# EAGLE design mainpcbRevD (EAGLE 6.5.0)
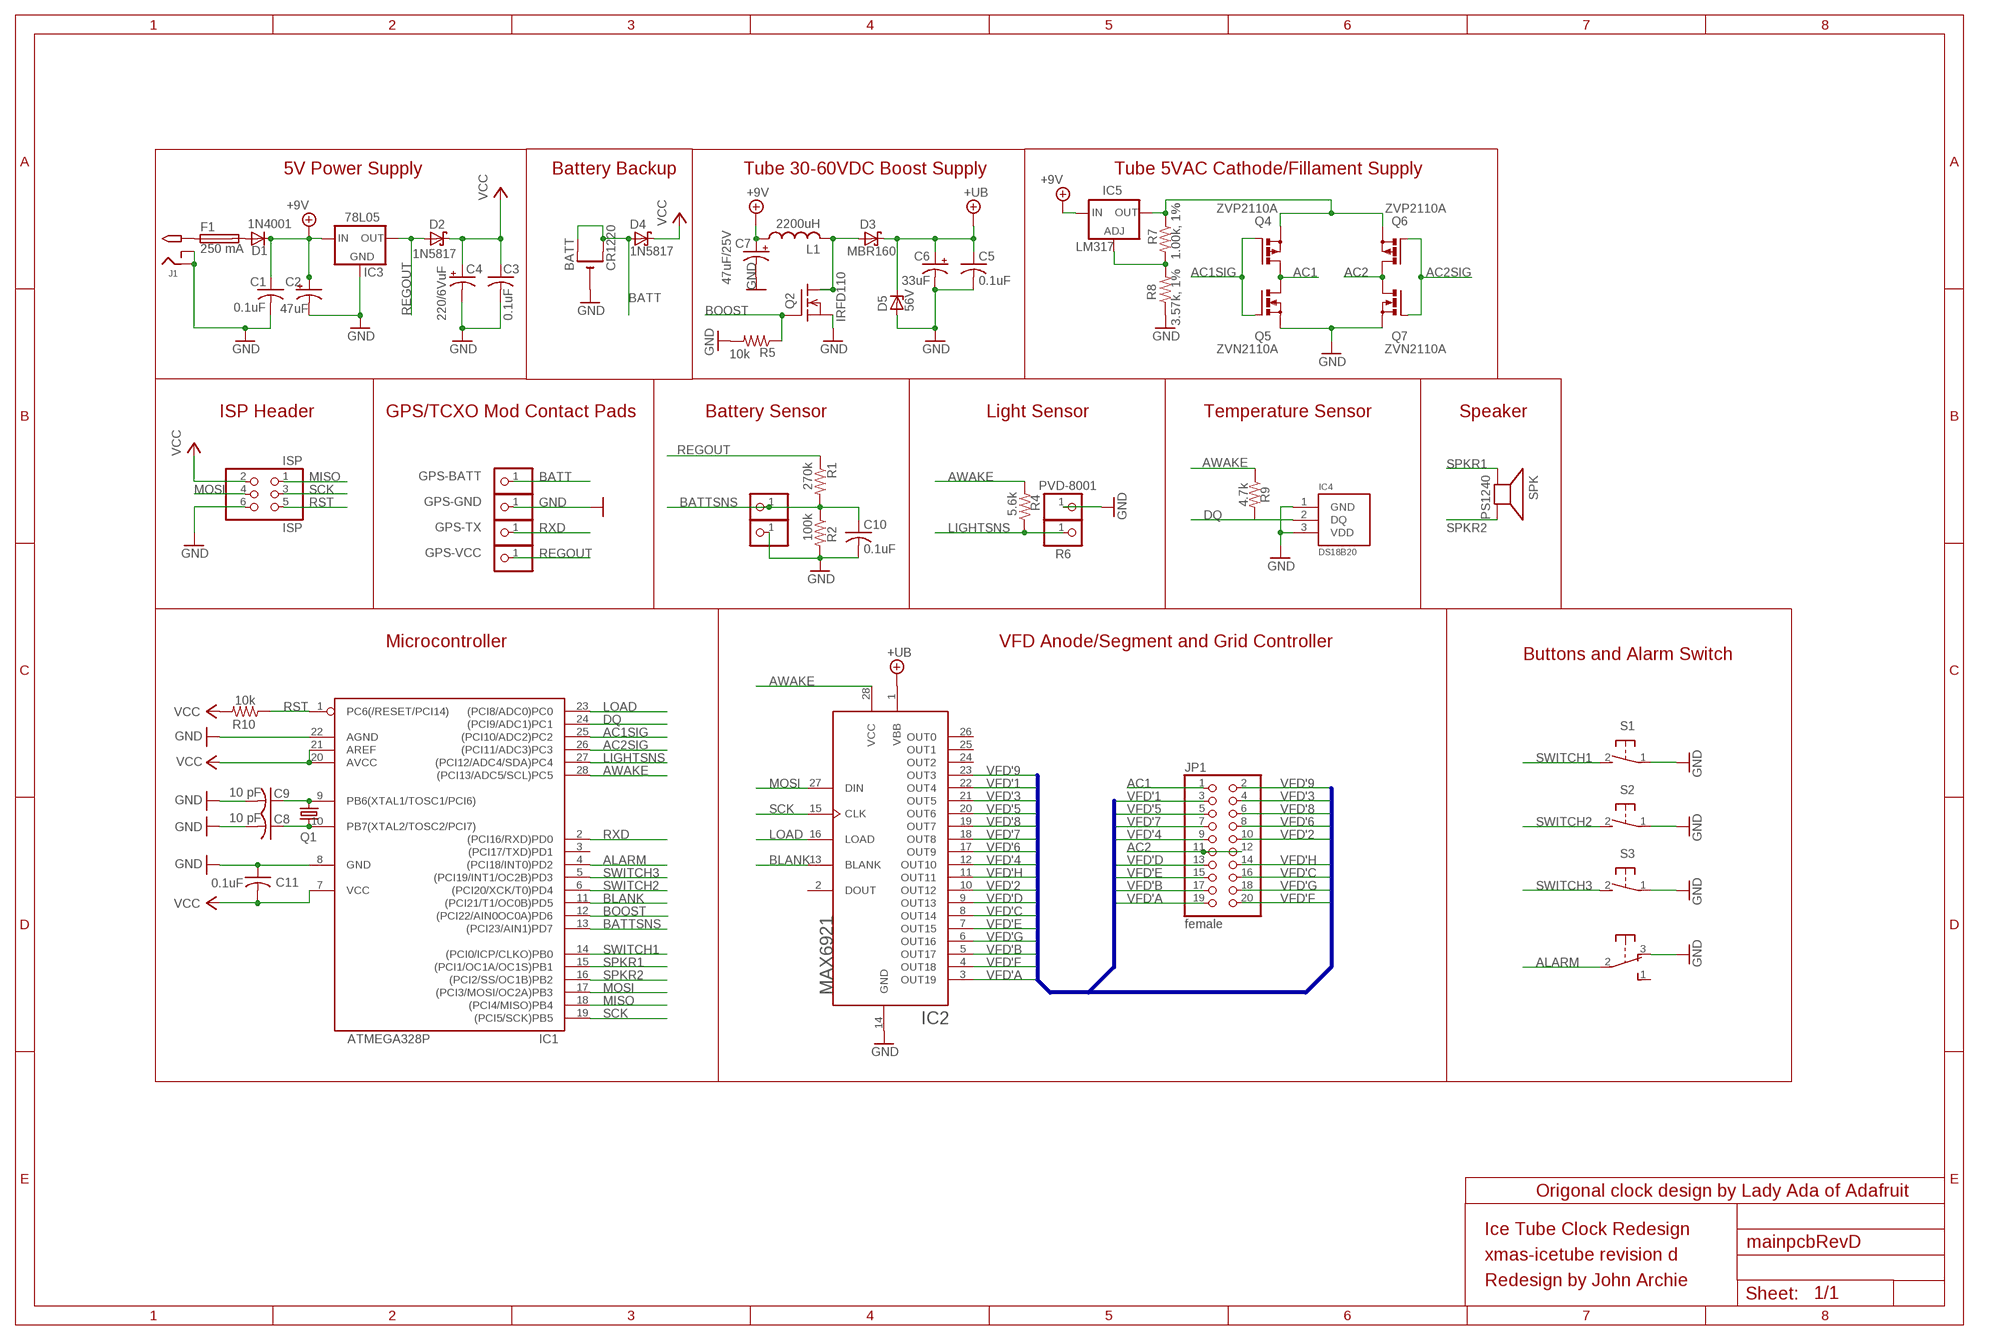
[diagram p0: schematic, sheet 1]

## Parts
BATT  CR1220  CR1220THM  [CR1220-THM]
C1  0.1uF  C-US025-025X050  [C025-025X050]
C2  47uF  CPOL-USE2.5-6  [E2,5-6]
C3  0.1uF  C-US025-025X050  [C025-025X050]
C4  220/6VuF  CPOL-USE2.5-6  [E2,5-6]
C5  0.1uF  C-US025-024X044  [C025-024X044]
C6  33uF  CPOL-USE3.5-8  [E3,5-8]
C7  47uF/25V  CPOL-USE2.5-6  [E2,5-6]
C8  10 pF  C-US025-024X044  [C025-024X044]
C9  10 pF  C-US025-024X044  [C025-024X044]
C10  0.1uF  C-US025-024X044  [C025-024X044]
C11  0.1uF  C-US025-025X050  [C025-025X050]
CT2  PINHD-1X1  [1X01]
CT3  PINHD-1X1  [1X01]
D1  1N4001  1N4004  [DO41-10]
D2  1N5817  SCHOTTKY-DIODEDO41  [DO41-10]
D3  MBR160  SCHOTTKY-DIODEDO41  [DO41-10]
D4  1N5817  SCHOTTKY-DIODEDO41  [DO41-10]
D5  56V  ZENER-DIODEDO41Z10  [DO41Z10]
F1  250 mA  FUSETE5  [TE5]
GPS-BATT  PINHD-1X1  [1X01]
GPS-GND  PINHD-1X1  [1X01]
GPS-TX  PINHD-1X1  [1X01]
GPS-VCC  PINHD-1X1  [1X01]
IC1  ATMEGA328P  ATMEGA168PROUND  [DIL28/3]
IC2  MAX6921  [PLCC-S28]
IC3  78L05  [TO92-LINE]
IC4  DS18B20  [TO92]
IC5  LM317  [TO92-LINE]
ISP  ISP  PINHD-2X3  [2X03]
J1  2.1MMJACK  [PJ-102A]
JP1  female  PINHD-2X10  [2X10]
L1  2200uH  L  [6000]
Q1  32.768 khz  CRYTALTC26V  [TC26V]
Q2  IRFD110  [DIL04]
Q4  ZVP2110A  [TO92-FLAT]
Q5  ZVN2110A  [TO92-FLAT]
Q6  ZVP2110A  [TO92-FLAT]
Q7  ZVN2110A  [TO92-FLAT]
R1  270k  R-US_0207/10  [0207/10]
R2  100k  R-US_0207/10  [0207/10]
R4  5.6k  R-US_0207/5V  [0207/5V]
R5  10k  R-US_0207/5V  [0207/5V]
R6  PVD-8001  PINHD-1X1  [1X01]
R6.1  PINHD-1X1  [1X01]
R7  1.00k, 1%  R-US_0207/5V  [0207/5V]
R8  3.57k, 1%  R-US_0207/5V  [0207/5V]
R9  4.7k  R-US_0207/10  [0207/10]
R10  10k  R-US_0207/5V  [0207/5V]
S1  31-XX  [B3F-31XX]
S2  31-XX  [B3F-31XX]
S3  31-XX  [B3F-31XX]
SPK  PS1240  SPEAKER/PS12  [PS12]
SW1  OS102011MA1Q  [OS102011MA1Q]

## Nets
+9V: C1.1 C2.+ C7.+ D1.C IC3.3(IN) IC5.3(IN) L1.1
+UB: C5.1 C6.+ D3.C D5.C IC2.1(VBB)
AC1: JP1.1 Q4.3(D) Q5.3(D)
AC1SIG: IC1.25((PCI10/ADC2)PC2) Q4.2(G) Q5.2(G)
AC2: JP1.11 JP1.12 Q6.3(D) Q7.3(D)
AC2SIG: IC1.26((PCI11/ADC3)PC3) Q6.2(G) Q7.2(G)
ALARM: IC1.4((PCI18/INT0)PD2) SW1.2(P)
AWAKE: IC1.28((PCI13/ADC5/SCL)PC5) IC2.28(VCC) R4.2 R9.1
BATT: BATT.+1(+) BATT.+2(+1) D4.A GPS-BATT.1
BATTSNS: C10.1 CT2.1 IC1.13((PCI23/AIN1)PD7) R1.2 R2.1
BLANK: IC1.11((PCI21/T1/OC0B)PD5) IC2.13(BLANK)
BOOST: IC1.12((PCI22/AIN0OC0A)PD6) Q2.3(G) R5.1
DQ: IC1.24((PCI9/ADC1)PC1) IC4.2(DQ) R9.2
GND: BATT.- C1.2 C2.- C3.2 C4.- C5.2 C6.- C7.- C8.2 C9.2 C10.2 C11.1 CT3.1 D5.A GPS-GND.1 IC1.8(GND) IC1.22(AGND) IC2.14(GND) IC3.2(GND) IC4.1(GND) IC4.3(VDD) ISP.6 J1.RING J1.RING_SW Q2.4(S) Q5.1(S) Q7.1(S) R2.2 R5.2 R6.1 R8.1 S1.1(P) S2.1(P) S3.1(P) SW1.3(O)
LIGHTSNS: IC1.27((PCI12/ADC4/SDA)PC4) R4.1 R6.1.1
LOAD: IC1.23((PCI8/ADC0)PC0) IC2.16(LOAD)
MISO: IC1.18((PCI4/MISO)PB4) ISP.1
MOSI: IC1.17((PCI3/MOSI/OC2A)PB3) IC2.27(DIN) ISP.4
N$1: C9.1 IC1.9(PB6(XTAL1/TOSC1/PCI6)) Q1.2
N$2: D3.A L1.2 Q2.1(D) Q2.2(D1)
N$3: C8.1 IC1.10(PB7(XTAL2/TOSC2/PCI7)) Q1.1
N$4: F1.1 J1.TIP
N$5: D1.A F1.2
N$6: IC5.1(ADJ) R7.2 R8.2
N$14: IC5.2(OUT) Q4.1(S) Q6.1(S) R7.1
REGOUT: D2.A GPS-VCC.1 IC3.1(OUT) R1.1
RST: IC1.1(PC6(/RESET/PCI14)) ISP.5 R10.1
RXD: GPS-TX.1 IC1.2((PCI16/RXD)PD0)
SCK: IC1.19((PCI5/SCK)PB5) IC2.15(CLK) ISP.3
SPKR1: IC1.15((PCI1/OC1A/OC1S)PB1) SPK.P$1(+)
SPKR2: IC1.16((PCI2/SS/OC1B)PB2) SPK.P$2(-)
SWITCH1: IC1.14((PCI0/ICP/CLKO)PB0) S1.2(S)
SWITCH2: IC1.6((PCI20/XCK/T0)PD4) S2.2(S)
SWITCH3: IC1.5((PCI19/INT1/OC2B)PD3) S3.2(S)
VCC: C3.1 C4.+ C11.2 D2.C D4.C IC1.7(VCC) IC1.20(AVCC) IC1.21(AREF) ISP.2 R10.2
VFD'1: IC2.22(OUT4) JP1.3
VFD'2: IC2.10(OUT12) JP1.10
VFD'3: IC2.21(OUT5) JP1.4
VFD'4: IC2.12(OUT10) JP1.9
VFD'5: IC2.20(OUT6) JP1.5
VFD'6: IC2.17(OUT9) JP1.8
VFD'7: IC2.18(OUT8) JP1.7
VFD'8: IC2.19(OUT7) JP1.6
VFD'9: IC2.23(OUT3) JP1.2
VFD'A: IC2.3(OUT19) JP1.19
VFD'B: IC2.5(OUT17) JP1.17
VFD'C: IC2.8(OUT14) JP1.16
VFD'D: IC2.9(OUT13) JP1.13
VFD'E: IC2.7(OUT15) JP1.15
VFD'F: IC2.4(OUT18) JP1.20
VFD'G: IC2.6(OUT16) JP1.18
VFD'H: IC2.11(OUT11) JP1.14
Unconnected: IC1.3((PCI17/TXD)PD1) IC2.2(DOUT) IC2.24(OUT2) IC2.25(OUT1) IC2.26(OUT0) SW1.1(S) SW1.MT1(MT) SW1.MT2(MT)

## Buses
VFD'[1..9],VFD'_A,VFD'_B,VFD'_C,VFD'_D,VFD'_E,VFD'_F,VFD'_G,VFD'_H

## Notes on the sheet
- 5V Power Supply | Battery Backup | Tube 30-60VDC Boost Supply | Tube 5VAC Cathode/Fillament Supply
- ISP Header | GPS/TCXO Mod Contact Pads | Battery Sensor | Light Sensor | Temperature Sensor | Speaker
- Microcontroller | VFD Anode/Segment and Grid Controller
- Buttons and Alarm Switch
- Origonal clock design by Lady Ada of Adafruit
- Ice Tube Clock Redesign
- xmas-icetube revision d
- Redesign by John Archie

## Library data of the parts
BATT = vfd:CR1220
C1 C3 C11 = minimidi:C-US: CAPACITOR, American symbol
C2 C4 C7 = minimidi:CPOL-US: POLARIZED CAPACITOR, American symbol
C5 C10 = rcl-ez:C-US: CAPACITOR, American symbol
C6 = rcl-ez:CPOL-US: POLARIZED CAPACITOR, American symbol
C8 C9 = resistor:C-US: CAPACITOR, American symbol
CT2 CT3 GPS-BATT GPS-GND GPS-TX GPS-VCC R6 R6.1 = ybox2:PINHD-1X1: PIN HEADER
D1 = minimidi:1N4004: DIODE
D2-D4 = usbbuck:SCHOTTKY-DIODE: Schottky Diode
D5 = diode:ZENER-DIODE: Z-Diode
F1 = fuse:FUSE: Fuse
IC1 = avr:ATMEGA168*P: MICROCONTROLLER 16 kBytes FLASH 1 kBytes SRAM 512 Bytes EEPROM USART 8-channel 10 bit ADC
IC2 = vfd:MAX6921
IC3 = jarchie:78L05
IC4 = jarchie:DS18B20
IC5 = jarchie:LM317: VOLTAGE REGULATOR
ISP = pinhead-ez:PINHD-2X3: PIN HEADER
J1 = minimidi:2.1MMJACK
JP1 = pinhead:PINHD-2X10: PIN HEADER
L1 = usbbuck:L
Q1 = crystal:CRYTAL: CRYSTAL
Q2 = vfd:IRFD110
Q4 Q6 = jarchie:ZVP2110A
Q5 Q7 = jarchie:ZVN2110A
R1 R2 R4 R5 R7-R10 = minimidi:R-US_: RESISTOR, American symbol
S1-S3 = switch-omron:31-XX: OMRON SWITCH
SPK = ybox2:SPEAKER: SPEAKER
SW1 = adaprog:OS102011MA1Q

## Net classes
0 default: clearance 0.205 mm

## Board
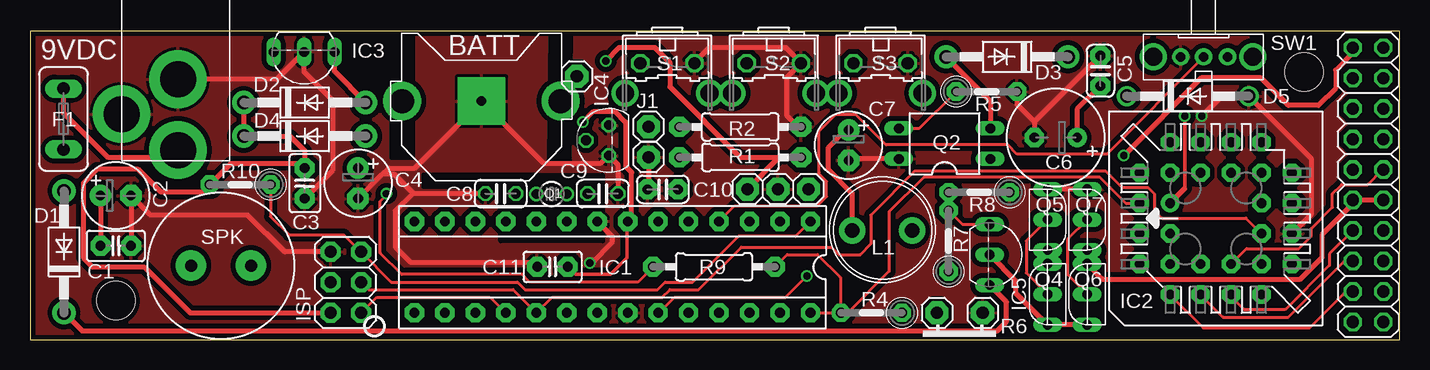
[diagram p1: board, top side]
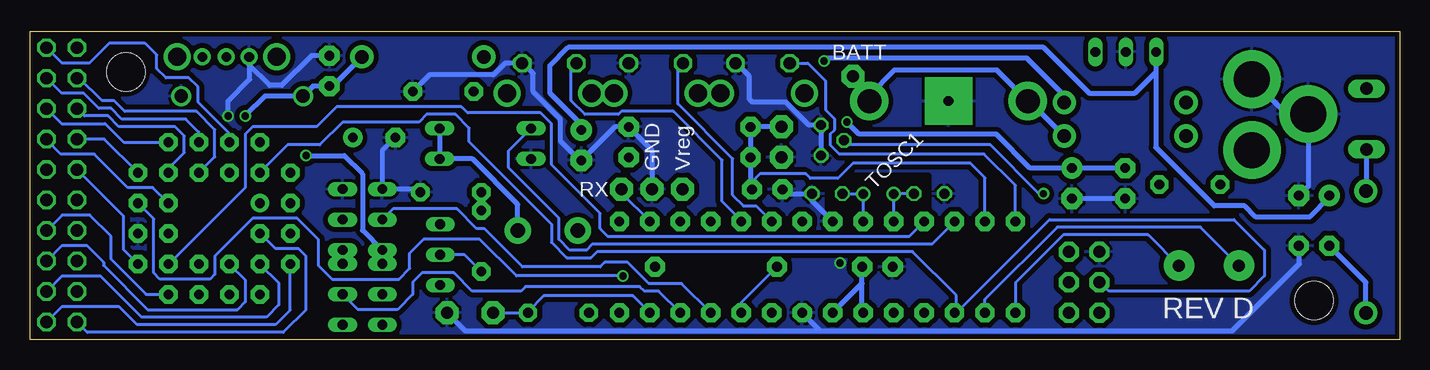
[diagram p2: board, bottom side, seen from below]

Size 114.2 x 25.71 mm. Coordinates in mm from the lower left corner, seen from the top.
Outline: 0,0 114.2,0 114.2,25.71 0,25.71 0,0
Copper layers (1*16): Top 0.0356mm / dielectric 1.5011mm / Bottom 0.0356mm
Design rules "LaenPCBOrder": minimum track width 6mil, minimum drill 13mil, track to track 6mil, track to pad 6mil, pad to pad 6mil, via to via 6mil, smd to smd 6mil, copper to edge 15mil, drill to drill 6mil, minimum pad ring 7mil, minimum via ring 7mil, stop-mask expansion 4mil, vias tented up to drill 0mil, thermal gap 10mil
Holes 3.2 mm at 106.21,22.31 7.15,3.26

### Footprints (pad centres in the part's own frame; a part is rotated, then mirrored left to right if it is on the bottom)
CR1220-THM = drill 2 pad 3.175: +1 -6.604,0; +2 6.604,0 | drill 0.8 pad 3.962 square: - 0,0
C025-025X050 = drill 0.813 pad 1.676 octagon: 1 -1.27,0; 2 1.27,0
E2,5-6 = drill 0.813 pad 1.778: + -1.27,0 | drill 0.813 pad 1.778 octagon: - 1.27,0
C025-024X044 = drill 0.813 pad 1.676 octagon: 1 -1.27,0; 2 1.27,0
E3,5-8 = drill 0.813 pad 1.6: + -1.778,0 | drill 0.813 pad 1.6 octagon: - 1.778,0
C025-024X044' = drill 0.813 octagon: 1 -1.27,0; 2 1.27,0
1X01 = drill 1.016 pad 1.93 octagon: 1 0,0
DO41-10 = drill 1.118 pad 1.93: A 5.08,0; C -5.08,0
DO41Z10 = drill 1.118: A 5.08,0; C -5.08,0
TE5 = drill 1.016 long: 1 -2.54,0; 2 2.54,0
DIL28/3 = drill 0.813 pad 1.6 octagon: 1 -16.51,-3.81; 2 -13.97,-3.81; 3 -11.43,-3.81; 4 -8.89,-3.81; 5 -6.35,-3.81; 6 -3.81,-3.81; 7 -1.27,-3.81; 8 1.27,-3.81; 9 3.81,-3.81; 10 6.35,-3.81; 11 8.89,-3.81; 12 11.43,-3.81; 13 13.97,-3.81; 14 16.51,-3.81; 15 16.51,3.81; 16 13.97,3.81; 17 11.43,3.81; 18 8.89,3.81; 19 6.35,3.81; 20 3.81,3.81; 21 1.27,3.81; 22 -1.27,3.81; 23 -3.81,3.81; 24 -6.35,3.81; 25 -8.89,3.81; 26 -11.43,3.81; 27 -13.97,3.81; 28 -16.51,3.81
PLCC-S28 = drill 0.813 pad 1.524: 1 1.27,3.81 | drill 0.813 pad 1.524 octagon: 2 -1.27,6.35; 3 -1.27,3.81; 4 -3.81,6.35; 5 -6.35,3.81; 6 -3.81,3.81; 7 -6.35,1.27; 8 -3.81,1.27; 9 -6.35,-1.27; 10 -3.81,-1.27; 11 -6.35,-3.81; 12 -3.81,-6.35; 13 -3.81,-3.81; 14 -1.27,-6.35; 15 -1.27,-3.81; 16 1.27,-6.35; 17 1.27,-3.81; 18 3.81,-6.35; 19 6.35,-3.81; 20 3.81,-3.81; 21 6.35,-1.27; 22 3.81,-1.27; 23 6.35,1.27; 24 3.81,1.27; 25 6.35,3.81; 26 3.81,6.35; 27 3.81,3.81; 28 1.27,6.35
TO92-LINE = drill 0.813 long: 1 -2.54,0; 2 0,0; 3 2.54,0
TO92 = drill 0.813 octagon: 1 1.27,0; 2 0,1.905; 3 -1.27,0
2X03 = drill 1.016 pad 1.676 octagon: 1 -2.54,-1.27; 2 -2.54,1.27; 3 0,-1.27; 4 0,1.27; 5 2.54,-1.27; 6 2.54,1.27
PJ-102A = drill 3 pad 4.8: RING 0.1,-3.39; RING_SW -4.6,-6.29; TIP 0.1,-9.29
2X10 = drill 1.016 octagon: 1 -11.43,-1.27; 2 -11.43,1.27; 3 -8.89,-1.27; 4 -8.89,1.27; 5 -6.35,-1.27; 6 -6.35,1.27; 7 -3.81,-1.27; 8 -3.81,1.27; 9 -1.27,-1.27; 10 -1.27,1.27; 11 1.27,-1.27; 12 1.27,1.27; 13 3.81,-1.27; 14 3.81,1.27; 15 6.35,-1.27; 16 6.35,1.27; 17 8.89,-1.27; 18 8.89,1.27; 19 11.43,-1.27; 20 11.43,1.27
6000 = drill 1.2 pad 2.184: 1 -2.5,0; 2 2.5,0
TC26V = drill 0.813: 1 -1.27,0; 2 1.27,0
DIL04 = drill 0.813 long: 1 -1.27,-3.81; 2 1.27,-3.81; 3 1.27,3.81; 4 -1.27,3.81
TO92-FLAT = drill 0.813 long: 1 -2.54,0; 2 0,0; 3 2.54,0
0207/10 = drill 0.813 pad 1.676 octagon: 1 -5.08,0; 2 5.08,0
0207/5V = drill 0.813 pad 1.524 octagon: 1 -2.54,0; 2 2.54,0
B3F-31XX = drill 1.016 octagon: 1 -2.261,-1.245; 2 2.261,-1.245 | drill 1.499 pad 2.159: 3 -3.505,1.245; 4 3.505,1.245
PS12 = drill 1 pad 2.54: P$1 -2.5,0; P$2 2.5,0
OS102011MA1Q = drill 0.8 pad 1.422: 1 -2,0; 2 0,0; 3 1.9,0 | drill 1.5 pad 2.184: MT1 -4.1,0; MT2 4.2,0

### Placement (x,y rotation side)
BATT  37.63,19.9 0 top
C1  7.15,7.84 0 top
C2  7.15,12.03 0 top
C3  22.9,13.04 270 top
C4  27.35,13.04 270 top
C5  89.24,22.41 90 top
C6  85.51,16.85 180 top
C7  68.24,16.22 270 top
C8  10 pF  [C025-024X044']  39.24,12.18 180 top
C9  10 pF  [C025-024X044']  47.75,12.18 0 top
C10  52.75,12.53 180 top
C11  43.56,6.08 0 top
CT2  51.56,17.77 0 top
CT3  51.56,15.23 0 top
D1  2.84,7.33 90 top
D2  22.9,19.77 0 top
D3  81.45,23.58 180 top
D4  22.9,16.98 0 top
D5  96.52,20.31 0 top
F1  2.79,18.4 270 top
GPS-BATT  45.59,21.96 0 top
GPS-GND  62.35,12.56 0 top
GPS-TX  64.89,12.56 0 top
GPS-VCC  59.81,12.56 0 top
IC1  48.56,6.06 180 top
IC2  98.85,10.12 90 top
IC3  22.86,23.99 180 top
IC4  48.25,16.62 90 top
IC5  80.01,7.1 270 top
ISP  26.33,4.79 90 top
J1  12.23,25.11 0 top
JP1  111.55,12.92 270 top
L1  71.04,9.11 0 top
Q1  43.48,12.15 0 top
Q2  76.24,16.35 90 top
Q4  84.83,3.8 90 top
Q5  84.83,10.02 270 top
Q6  88.13,3.8 90 top
Q7  88.13,10.02 270 top
R1  59.21,15.2 180 top
R2  59.21,17.74 0 top
R4  70.15,2.25 180 top
R5  79.75,20.69 0 top
R6  79.42,2.25 0 top
R6.1  75.61,2.25 0 top
R7  76.58,8.24 90 top
R8  79.12,12.31 180 top
R9  57.02,6.08 180 top
R10  17.52,12.94 180 top
S1  53.13,21.81 180 top
S2  62.02,21.81 180 top
S3  70.91,21.81 180 top
SPK  15.92,6.19 180 top
SW1  97.83,23.58 180 top

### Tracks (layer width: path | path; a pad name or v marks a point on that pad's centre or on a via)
+9V
  Top 0.406: C2.+ C1.1 | L1.1 68.54,12.22 66.54,14.21 66.54,15.99 68.04,17.49 C7.+ | D1.C 4.33,0.75 80.64,0.75 81.4,1.51 81.4,3.16 IC5.3
  Bottom 0.406: 20.32,22.34 22.09,20.56 25.9,20.56 29.71,24.37 69.34,24.37 70.86,22.85 70.86,20.56 68.24,17.94 C7.+ | D1.C 2.84,4.79 C1.1 | C2.+ 5.88,11.88 7.49,10.27 12.06,10.27 12.95,11.16 15.49,11.16 20.36,16.04 20.32,16.08 20.32,22.34 | 20.32,22.34 IC3.3
+UB  (via drill 0.6)
  Top 0.305: v96.26,18.66 96.26,12.62
  Top 0.406: 96.26,12.62 IC2.1 | C5.1 87.29,19.2 C6.+
  Bottom 0.406: v96.26,18.66 94.61,20.31 D5.C 90.6,21.14 C5.1 88.97,21.14 D3.C
AC1  (via drill 0.6)
  Top 0.406: v91.18,15.35 97.66,21.83 102.61,21.83 104.9,19.55 107.44,19.55 108.83,20.94 108.83,22.47 110.28,23.91 JP1.1 | Q4.3 Q5.3
  Bottom 0.406: v91.18,15.35 88.01,15.35 86.48,13.83 86.48,9.13 Q5.3
AC1SIG
  Top 0.254: Q5.2 83.05,8.24 83.05,5.58 Q4.2
  Bottom 0.254: Q5.2 83.94,10.91 78.61,10.91 76.96,9.26 76.32,9.26 73.15,6.08 66.67,6.08 66.29,6.46 64.38,6.46 62.61,4.69 59.88,4.69 IC1.25
AC2
  Top 0.406: JP1.12 JP1.11 110.28,11.34 107.69,8.75 107.69,6.85 105.91,5.07 89.4,5.07 Q6.3 Q7.3
AC2SIG
  Top 0.254: Q7.2 86.48,8.37 86.48,5.45 Q6.2
  Bottom 0.254: IC1.26 61.79,4.05 62.99,4.05 63.37,4.43 72.89,4.43 73.27,4.05 77.34,4.05 78.86,5.58 81.53,5.58 82.29,4.81 82.29,3.8 83.56,2.53 86.86,2.53 Q6.2
ALARM
  Top 0.254: IC1.4 58.74,11.16 65.65,11.16 66.42,11.93 66.42,13.2 65.78,13.83 65.78,13.96 65.78,14.47 65.78,17.39 67.18,18.78 68.83,18.78 71.37,16.24 81.53,16.24 82.29,15.48 89.78,15.48 97.83,23.53 SW1.2
AWAKE
  Top 0.254: IC2.28 91.33,11.39 89.15,13.58 74.54,13.58 71.62,10.66 71.62,5.7 68.26,2.34 67.6,2.34 67.56,2.3 | 67.56,2.3 67.56,5.19 65.65,7.1 63.11,7.1 R9.1 | IC1.28 R4.2 67.56,2.3
BATT
  Bottom 0.406: D4.A 30.9,19.9 BATT.+1 33.59,22.47 42.16,22.47 44.24,20.39 | 44.24,20.39 BATT.+2 | GPS-BATT.1 44.24,20.61 44.24,20.39
BATTSNS
  Bottom 0.254: IC1.13 34.59,13.5 35.81,14.72 45.59,14.72 46.86,13.45 49.14,13.45 49.52,13.83 53.37,13.83 54.13,13.07 54.13,12.65
  Bottom 0.406: CT2.1 54.1,17.77 R2.1 R1.2 54.13,12.65 C10.1
BLANK
  Bottom 0.254: IC1.11 39.67,9.85 40.89,8.62 66.04,8.62 66.67,9.26 66.67,10.53 70.73,14.59 70.73,14.85 70.73,15.48 70.73,18.02 71.62,18.91 77.72,18.91 78.23,19.42 88.64,19.42 90.29,17.77 95.63,17.77 96.26,17.13 96.26,12.69 102.64,6.31 IC2.13
BOOST
  Top 0.254: Q2.3 74.14,17.62 R5.1
  Bottom 0.254: Q2.3 74.29,15.76 74.29,14.34 70.1,10.15 70.1,8.37 69.21,7.48 67.81,7.48 67.31,7.99 38.98,7.99 37.13,9.85 IC1.12
DQ  (via drill 0.6)
  Top 0.254: R9.2 50.67,4.81 41.65,4.81 41.02,5.45 30.98,5.45 29.21,7.23 29.21,11.54 29.71,12.05 v29.71,12.18
  Bottom 0.254: 46.1,16.37 IC4.2 45.97,16.24 34.16,16.24 30.09,12.18 v29.71,12.18 | R9.2 54.91,3.12 IC1.24
GND  (via drill 0.6)
  Top 0.406: IC2.14 106.8,10.46 106.8,15.1 D5.A 99.34,20.31 v97.69,18.66 | C1.2 C2.- 10.03,10.42 10.03,10.4 18.16,10.4 21.23,7.33 ISP.6 | 37.53,19.8 BATT.- | BATT.- 42.82,14.72 47.62,14.72 IC4.3 49.02,14.59 C9.2 | J1.RING 12.35,21.7 20.57,21.7 IC3.2 22.86,22.34 25.27,19.93 25.27,14.14 C3.2 | BATT.- 32.05,14.31 29.89,14.31 29.37,13.79 | C8.2 31.97,12.18 31.92,12.23 | C5.2 83.73,18.18 | R5.2 82.29,19.63 83.73,18.18 | CT3.1 51.56,12.62 C10.2 | S1.1 55.39,23.12 56.64,24.37 62.99,24.37 64.28,23.08 S2.1 63.11,21.89 63.11,18.66 64,17.77 64.26,17.77 R2.2 | C4.- 29.37,13.79 | 31.92,12.23 30.36,13.79 29.37,13.79 | C11.1 41.9,6.46 31.75,6.46 30.48,7.73 30.48,10.78 31.92,12.23 | IC1.8 48.51,8.65 48.51,8.12 46.79,6.4 v46.67,6.4 | Q2.4 68.37,15.08 C7.- | 83.73,18.18 C6.- | Q7.1 Q5.1
  Bottom 0.406: IC4.3 IC4.1 49.27,17.89 51.18,19.8 53.97,19.8 54.22,20.05 54.22,21.96 55.32,23.05 S1.1 | C5.2 90.73,23.68 93.21,21.2 94.23,21.2 95.93,22.9 SW1.3 95.88,23.53 95.88,21.7 97.69,19.9 v97.69,18.66 | 73.15,23.03 S3.1 | S3.1 74.59,23.05 75.56,22.09 80.89,22.09 R5.2 | J1.RING 9.43,18.82 J1.RING_SW 7.63,12.82 C2.- | IC1.8 49.02,11.6 C9.2 51.25,12.18 C10.2 | GPS-GND.1 62.35,15.81 R2.2 65.45,17.74 C7.- 68.37,14.95 69.97,16.55 69.97,18.4 72.26,20.69 72.26,22.21 73.1,23.05 S3.1 | IC1.22 48.33,0.75 | C3.2 C4.- | 48.33,0.75 13.96,0.75 8.38,6.34 8.38,7.79 C1.2 | C6.- 84.83,15.76 Q5.1 81.91,12.56 R8.1 | R6.1 77.92,0.75 48.33,0.75
  pour Bottom (isolate 0.406, rank 2): -0.01,25.64 -0.01,-0.01 114.17,-0.01 114.17,25.64
  pour Top (isolate 0.406, rank 2): -0.01,25.64 -0.01,-0.01 114.17,-0.01 114.17,25.64
LIGHTSNS
  Bottom 0.254: IC1.27 63.95,3.67 71.37,3.67 72.69,2.35 R4.1 R6.1.1
LOAD  (via drill 0.6)
  Top 0.254: IC1.23 52.42,2.25 53.72,3.54 62.99,3.54 v64.77,5.32
  Bottom 0.254: IC2.16 103.88,10.08 103.88,5.58 103.37,5.07 99.18,5.07 98.8,5.45 98.8,6.97 95.63,10.15 91.94,10.15 90.17,8.37 90.17,6.21 89.02,5.07 83.43,5.07 82.55,5.96 82.55,7.23 81.4,8.37 76.7,8.37 73.66,5.32 v64.77,5.32
MISO
  Top 0.254: IC1.18 39.64,2.25 38.35,3.54 28.9,3.54 ISP.1
MOSI
  Bottom 0.254: ISP.4 24.99,4.79 24.25,4.05 12.57,4.05 11.3,5.32 11.3,7.48 13.84,10.02 29.21,10.02 36.98,2.25 IC1.17 36.98,2.4 36.98,3.7 40.63,7.35 66.92,7.35 67.43,6.85 69.46,6.85 70.73,8.12 70.73,9.64 77.59,16.5 77.59,17.64 78.73,18.78 81.15,18.78 81.78,18.15 88.13,18.15 90.04,16.24 92.73,16.24 IC2.27
N$1
  Bottom 0.254: IC1.9 Q1.2 44.77,12.18 C9.1
N$2
  Top 0.406: D3.A 80.05,19.9 Q2.2
  Bottom 0.406: Q2.2 Q2.1 | 80.03,15.1 Q2.1 | L1.2 73.54,11.3 77.31,15.08 Q2.1
N$3
  Bottom 0.254: IC1.10 Q1.1 42.18,12.18 C8.1
N$4
  Top 0.406: F1.1 2.79,18.91 6.47,15.23 11.74,15.23 J1.TIP
N$5
  Bottom 0.406: F1.2 2.79,12.46 D1.A
N$6
  Top 0.254: R7.2 77.72,9.64 IC5.1
  Bottom 0.254: R8.2 R7.2
N$9
  cutout Top: 30.09,25.64 32,25.64 32,15.1 30.09,15.1
N$14
  Top 0.406: IC5.2 82.16,4.94 82.16,3.92 Q4.1 Q6.1
  Bottom 0.254: R7.1 77.97,7.1 IC5.2
N$18
  cutout Bottom: 39.24,8.24 39.24,13.7 47.75,13.7 47.75,8.24
N$19
  cutout Top: 39.24,13.7 47.75,13.7 47.75,8.24 39.24,8.24
N$21
  cutout Top: 32.76,13.83 42.29,13.83 42.29,12.69 32.76,12.69
N$23
  cutout Top: 43.3,25.64 43.17,14.97 45.08,14.97 45.21,25.64
REGOUT  (via drill 0.6)
  Top 0.406: D2.A 25.39,22.36 IC3.1 | v48,23.23 49.14,24.37 52.06,24.37 53.34,23.1 53.34,21.07 59.2,15.2 R1.1 62.45,15.2 GPS-VCC.1
  Bottom 0.406: D2.A 27.98,20.35 31.11,23.48 47.75,23.48 v48,23.23
RST
  Top 0.254: IC1.1 63.82,8.62 59.05,8.62 55.24,4.81 52.95,4.81 52.32,4.18 41.27,4.18 40.63,4.81 30.12,4.81 ISP.5 27.58,7.33 26.16,8.75 21.59,8.75 20.06,10.27 R10.1
RXD
  Bottom 0.254: IC1.2 64.89,12.23 GPS-TX.1
SCK
  Top 0.254: ISP.3 28.21,4.18 40.28,4.18 IC1.19 43.5,3.54 52.7,3.54 53.34,4.18 55.75,4.18 59.3,7.73 66.8,7.73 67.43,7.1 69.21,7.1 70.1,7.99 70.1,10.4 73.78,14.08 89.66,14.08 89.78,13.96 90.1,13.64 91.05,12.69 93.21,12.69 93.72,12.18 93.72,10.78 94.36,10.15 101.36,10.15 IC2.15
SPKR1
  Bottom 0.254: IC1.15 32.05,4.77 28.06,8.75 20.98,8.75 SPK.P$1
SPKR2
  Bottom 0.254: IC1.16 34.59,3.37 28.57,9.39 16.76,9.39 16.62,9.39 SPK.P$2
SWITCH1
  Bottom 0.254: S1.2 49.35,23.05 47.87,21.58 47.87,19.16 47.11,18.4 47.11,17.51 47.49,17.13 47.49,16.24 46.73,15.48 34.67,15.48 32.05,12.86 IC1.14
SWITCH2
  Bottom 0.254: IC1.6 53.66,11.16 54.73,11.16 55.62,12.05 55.62,15.1 60.19,19.67 60.19,22.62 S2.2
SWITCH3
  Bottom 0.254: IC1.5 54.91,9.94 56.51,11.54 56.51,14.97 60.57,19.04 64.89,19.04 65.14,18.79 67.93,18.79 69.08,19.94 69.08,22.62 S3.2
VCC  (via drill 0.6)
  Top 0.305: 49.78,9.89 49.78,6.85 48.38,5.45 45.46,5.45 C11.2
  Top 0.406: D2.C D4.C 21.71,16.98 22.92,15.77 C3.1 22.9,14.33 22.52,14.71 16.75,14.71 R10.2 14.35,12.31 10.92,12.31 9.01,14.21 5.58,14.21 4.44,13.07 4.44,6.85 5.2,6.08 9.52,6.08 13.35,2.25 ISP.2 | v46.1,18.15 46.98,19.04 48.76,19.04 49.65,18.15 49.65,14.47 50.16,13.96 50.16,10.2 IC1.7 49.8,9.87 49.78,9.89
  Bottom 0.406: v46.1,18.15 45.08,17.13 33.65,17.13 30.83,14.31 C4.+ C3.1 | IC1.20 44.83,2.33 C11.2 44.83,4.71 IC1.21
VFD'1
  Bottom 0.254: 110.21,21.81 JP1.3 110.08,21.81 108.2,19.93 107.18,19.93 106.29,19.04 100.33,19.04 98.8,17.51 98.8,15.25 IC2.22
VFD'2
  Top 0.254: IC2.10 101.41,7.61 105.79,7.61 106.8,8.62 106.8,9.26 108.58,11.04 108.58,12.18 109.34,12.94 111.5,12.94 112.75,14.19 JP1.10
VFD'3
  Bottom 0.254: IC2.21 100.12,17.31 101.21,18.4 106.55,18.4 107.44,19.29 108.45,19.29 109.72,20.56 111.57,20.56 JP1.4
VFD'4
  Bottom 0.254: JP1.9 106.42,10.33 106.42,7.54 IC2.12
VFD'5
  Bottom 0.254: IC2.20 102.66,14.29 101.34,15.61 101.34,17.01 102.1,17.77 106.8,17.77 107.69,18.66 109.67,18.66 JP1.5
VFD'6
  Bottom 0.254: IC2.17 103.95,12.69 106.04,12.69 108.83,15.48 111.63,15.48 112.82,16.67 JP1.8
VFD'7
  Bottom 0.254: IC2.18 107.99,16.73 JP1.7
VFD'8
  Bottom 0.254: JP1.6 111.57,18.02 107.95,18.02 106.4,16.47 IC2.19
VFD'9
  Bottom 0.254: JP1.2 111.57,23.1 109.22,23.1 107.56,24.75 104.64,24.75 103.63,23.74 103.63,22.59 102.87,21.83 100.96,21.83 100.2,21.07 100.2,19.8 97.53,17.13 97.53,16.52 IC2.23
VFD'A
  Bottom 0.254: JP1.19 109.41,0.62 93.09,0.62 91.18,2.53 91.18,6.97 91.82,7.61 93.72,7.61 94.97,8.85 IC2.3
VFD'B
  Top 0.254: IC2.5 97.81,1 106.68,1 109.7,4.03 JP1.17
VFD'C
  Bottom 0.254: JP1.16 111.52,7.86 109.47,7.86 108.07,6.46 108.07,6.21 104.39,2.53 96.9,2.53 96.26,3.16 96.26,5 IC2.8
VFD'D
  Top 0.254: JP1.13 108.33,7.15 108.33,6.21 104.64,2.53 101.21,2.53 100.12,3.62 IC2.9
VFD'E
  Top 0.254: IC2.7 99.46,1.89 104.9,1.89 109.57,6.57 JP1.15
VFD'F
  Bottom 0.254: JP1.20 111.52,2.78 106.8,2.78 105.28,1.26 93.72,1.26 92.5,2.48 IC2.4
VFD'G
  Bottom 0.254: JP1.18 111.52,5.32 108.33,5.32 104.9,1.89 94.48,1.89 93.47,2.91 93.47,4.74 IC2.6
VFD'H
  Bottom 0.254: JP1.14 111.52,10.4 109.22,10.4 107.44,8.62 107.44,6.72 104.52,3.8 102.68,3.8 IC2.11

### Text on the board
tNames: 9VDC | J1
bNames: BATT | Vreg | GND | TOSC1 | RX
_bsilk: REV D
